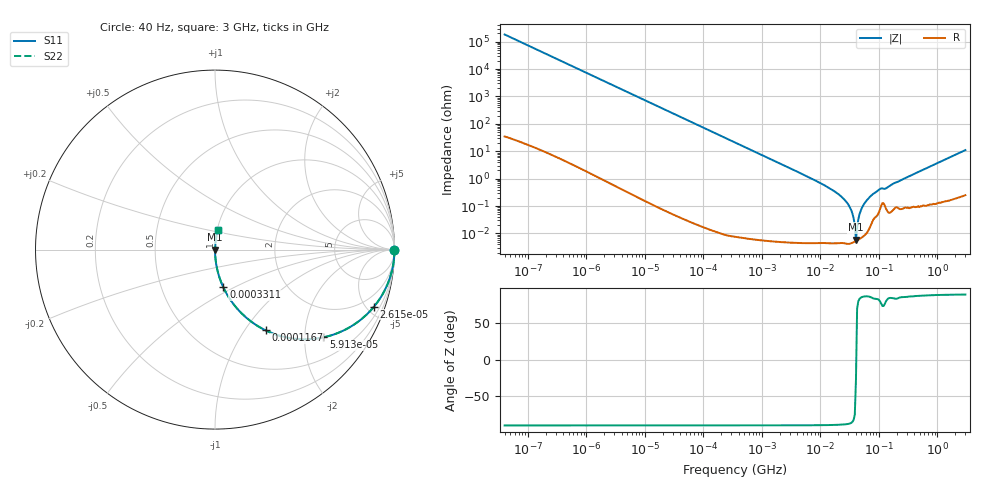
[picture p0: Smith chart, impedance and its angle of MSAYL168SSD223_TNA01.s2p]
! MSAYL168SSD223_TNA01  S-PARAMETER MODEL  ( General Type )
! Model Generated by TAIYO YUDEN Corporation (http://www.ty-top.com)
! Version 2.0
! TAIYO YUDEN Control No. 030711
! Copyright(c) 2003 TAIYO YUDEN CO.,LTD. All Rights Reserved.
! Product Description (link to TY-COMPAS)
! https://ds.yuden.co.jp/TYCOMPAS/or/detail?pn=MSAYL168SSD223KTNA01&u=M
! Products Name : Multilayer Ceramic Capacitors
! Characteristics :
!  Capacitance : 0.022 uF , Rated Voltage : 10V
!  Case Size : 1.6 x 0.8 / 0.063 x 0.031 [mm/inch] , Thickness : 0.8 / 0.031 [mm/inch]
!  (Conditions: Temperature = 25 degC , DC Bias Current/Voltage = 0A / 0V)
! External Node Assignments :
!  1  o---| |---o  2
! GND o---------o GND
! Frequency Range : 40Hz  -  3GHz  [ 401 STEP ]
# MHz S RI R 50
! Freq[MHz].  S11 Real  S11 Imag  S21 Real  S21 Imag  S12 Real  S12 Imag  S22 Real  S22 Imag
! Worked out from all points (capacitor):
!   401 points, 40 Hz to 3 GHz, reference 50 ohm
!   read as one part in series: C = 21.8 nF near 44 Hz
!   lowest |Z| = 6.03 mohm at 40.44 MHz (marker M1)
!   series resonance near 40.74 MHz, so ESL is about 700 pH
!   S11 on the Smith chart (normalised r, x): 40 Hz: open; 26.14 kHz: 1.00, -5.59; 59.12 kHz: 1.00, -2.47; 116.7 kHz: 1.00, -1.25; 331.1 kHz: 1.00, -0.44; 3 GHz: 1.01, +0.22
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4e-05  1 -0.000548  4.04e-07 0.000548  4.04e-07 0.000548  1 -0.000548
0.000834  0.9999 -0.0114  0.000133 0.0114  0.000133 0.0114  0.9999 -0.0114
0.005113  0.9951 -0.0697  0.00489 0.0697  0.00489 0.0697  0.9951 -0.0697
0.017386  0.9463 -0.2253  0.0537 0.2253  0.0537 0.2253  0.9463 -0.2253
0.026145  0.8863 -0.3173  0.1137 0.3173  0.1137 0.3173  0.8863 -0.3173
0.059125  0.6039 -0.489  0.3961 0.489  0.3961 0.489  0.6039 -0.489
0.116704  0.2814 -0.4495  0.7186 0.4495  0.7186 0.4495  0.2814 -0.4495
0.331057  0.0464 -0.2103  0.9536 0.2103  0.9536 0.2103  0.0464 -0.2103
0.362475  0.0391 -0.1935  0.9609 0.1935  0.9609 0.1935  0.0391 -0.1935
1.178032  0.00387 -0.0617  0.9961 0.0617  0.9961 0.0617  0.00387 -0.0617
7.222098  0.00014 -0.0098  0.9999 0.0098  0.9999 0.0098  0.00014 -0.0098
15.60822  5.95e-05 -0.004  0.9999 0.004  0.9999 0.004  5.95e-05 -0.004
24.56009  4.82e-05 -0.0019  1 0.0019  1 0.0019  4.82e-05 -0.0019
32.2371  4.33e-05 -0.000847  1 0.000847  1 0.000847  4.33e-05 -0.000847
38.64618  5.07e-05 -0.000189  0.9999 0.000189  0.9999 0.000189  5.07e-05 -0.000189
40.43842  5.32e-05 -2.83e-05  0.9999 2.83e-05  0.9999 2.83e-05  5.32e-05 -2.83e-05
44.27611  5.9e-05 0.000313  0.9999 -0.000313  0.9999 -0.000313  5.9e-05 0.000313
50.72622  7.17e-05 0.000829  0.9999 -0.000829  0.9999 -0.000829  7.17e-05 0.000829
63.63129  0.000117 0.00173  0.9999 -0.00173  0.9999 -0.00173  0.000117 0.00173
100.1261  0.000618 0.0039  0.9994 -0.0039  0.9994 -0.0039  0.000618 0.0039
150.5692  0.000595 0.00535  0.9994 -0.00535  0.9994 -0.00535  0.000595 0.00535
3000  0.0145 0.1086  0.9855 -0.1086  0.9855 -0.1086  0.0145 0.1086
